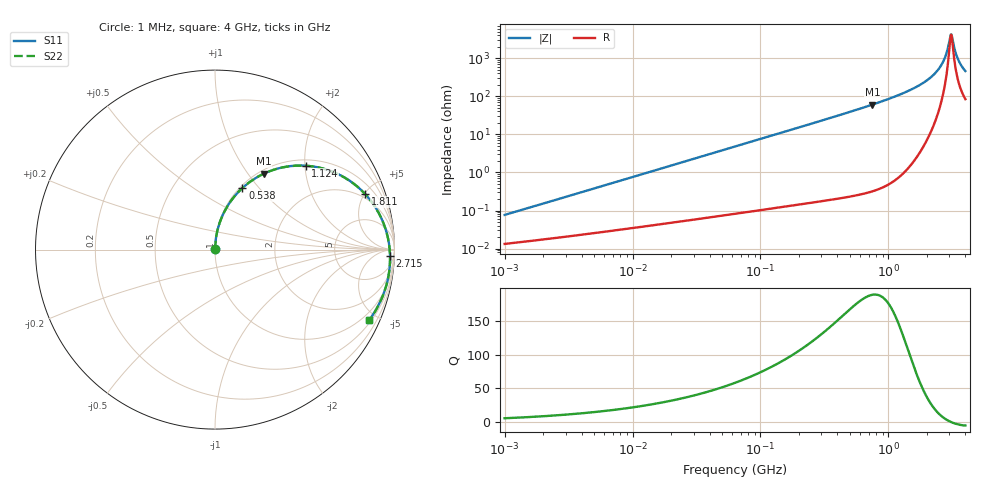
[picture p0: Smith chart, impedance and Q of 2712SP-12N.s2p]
# MHz  S  MA  R  50
!Freq  MagS11  AngS11  MagS21  AngS21  MagS12  AngS12  MagS22  AngS22
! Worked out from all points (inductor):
!   801 points, 1 MHz to 4 GHz, reference 50 ohm
!   read as one part in series: L = 12 nH near 1.042 MHz
!   highest Q = 189 at 749.9 MHz (marker M1), where L = 12.8 nH
!   self-resonance near 3.075 GHz
!   S11 on the Smith chart (normalised r, x): 1 MHz: 1.00, +0.00; 538 MHz: 1.03, +0.82; 1.124 GHz: 1.14, +2.01; 1.811 GHz: 1.67, +5.06; 2.715 GHz: 24, -37; 4 GHz: 0.62, -4.52
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1  0.0007424 79.6  0.9999 -0.0  0.9999 -0.0  0.0007424 79.6
4.016383  0.002943 85.3  0.9998 -0.2  0.9998 -0.2  0.002943 85.3
15.96482  0.01167 87.2  0.9995 -0.7  0.9995 -0.7  0.01166 87.2
63.45894  0.0463 86.1  0.9981 -2.8  0.9981 -2.8  0.0463 86.1
252.2445  0.1822 78.3  0.9817 -11.2  0.9817 -11.2  0.1822 78.3
537.993  0.3754 66.0  0.9246 -23.6  0.9246 -23.6  0.3753 66.0
749.8529  0.503 57.3  0.8616 -32.4  0.8616 -32.4  0.5029 57.3
1013.11  0.6386 47.0  0.7659 -42.7  0.7659 -42.7  0.6384 47.0
1123.878  0.6876 42.8  0.7218 -46.8  0.7218 -46.8  0.6873 42.8
1441.679  0.8022 31.8  0.5894 -57.7  0.5894 -57.7  0.8019 31.8
1811.364  0.8922 20.3  0.4353 -68.6  0.4353 -68.6  0.8919 20.3
2323.568  0.9578 6.7  0.2394 -80.2  0.2394 -80.2  0.9576 6.7
2524.674  0.9699 2.0  0.1707 -82.8  0.1707 -82.8  0.9698 2.0
2714.869  0.9761 -2.2  0.1106 -82.9  0.1106 -82.9  0.976 -2.2
2829.918  0.9778 -4.6  0.07702 -80.0  0.07702 -80.0  0.9778 -4.6
3011.696  0.9778 -8.2  0.03167 -54.8  0.03167 -54.8  0.978 -8.2
3106.919  0.9768 -10.0  0.02316 -3.9  0.02316 -3.9  0.977 -10.0
3205.151  0.975 -11.8  0.03685 36.8  0.03685 36.8  0.9753 -11.8
3375.823  0.9706 -14.8  0.07391 54.0  0.07391 54.0  0.971 -14.8
3518.882  0.9658 -17.2  0.1052 57.0  0.1052 57.0  0.9663 -17.2
3744.916  0.9566 -20.7  0.1514 57.1  0.1514 57.1  0.9573 -20.7
4000  0.9447 -24.5  0.1984 55.2  0.1984 55.2  0.9456 -24.5
